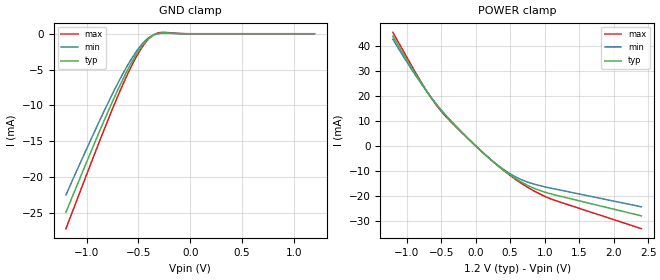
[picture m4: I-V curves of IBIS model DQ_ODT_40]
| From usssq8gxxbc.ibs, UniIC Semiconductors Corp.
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|   Model DQ_ODT_40
[Model] DQ_ODT_40
Model_type Input
Polarity   Non-Inverting
Enable   Active-High
Vinl =  8.300E-01
Vinh =  9.700E-01
C_comp   6.861E-13   6.852E-13   6.894E-13
C_comp_power_clamp   2.572E-13   2.550E-13   2.616E-13
C_comp_gnd_clamp   4.125E-13   4.123E-13   4.156E-13
[Model Spec]
Vinh   9.700E-01   9.250E-01   1.015E+00
Vinl   8.300E-01   7.850E-01   8.750E-01
[Temperature Range]   4.500E+01   9.500E+01   0.000E+00
[Voltage Range]   1.200E+00   1.140E+00   1.260E+00
[C Comp Corner]
C_comp_power_clamp   2.572E-13   2.616E-13   2.550E-13
C_comp_gnd_clamp   4.125E-13   4.123E-13   4.156E-13
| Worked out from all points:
|   GND clamp passes 1 mA (typ) near -0.42 V on its own axis
|   POWER clamp passes 1 mA (typ) near -0.04 V on its own axis
[GND_clamp]
|Voltage   I(typ)   I(min)   I(max)
-1.2V     -24.87mA   -22.47mA   -27.16mA
-875mV    -13.58mA   -12.11mA   -14.96mA
-750mV    -9.434mA   -8.354mA   -10.45mA
-650mV    -6.338mA   -5.564mA   -7.063mA
-575mV    -4.234mA   -3.679mA   -4.736mA
-500mV    -2.413mA   -2.066mA   -2.698mA
-425mV    -1.004mA   -845.7uA   -1.103mA
-375mV    -372.1uA   -318.3uA   -373.8uA
-325mV    -19.34uA   -35.56uA   45.93uA
-275mV    99.8uA     61.11uA    185.6uA
-25mV     0A         0A         0A
1.2V      0A         0A         0A
[POWER_clamp]
|Voltage   I(typ)   I(min)   I(max)
-1.2V     43.98mA    42.77mA    45.49mA
-1V       34.69mA    33.81mA    35.68mA
-775mV    24.66mA    24.42mA    24.89mA
-650mV    19.61mA    19.62mA    19.47mA
-525mV    15.11mA    15.24mA    14.76mA
-375mV    10.42mA    10.53mA    10.11mA
0V        32.96nA    74.84nA    14.75nA
225mV     -5.69mA    -5.607mA   -5.654mA
425mV     -10.17mA   -9.835mA   -10.25mA
700mV     -15.06mA   -13.96mA   -15.69mA
1.05V     -18.93mA   -16.7mA    -20.79mA
2.4V      -28.03mA   -24.4mA    -33.17mA
